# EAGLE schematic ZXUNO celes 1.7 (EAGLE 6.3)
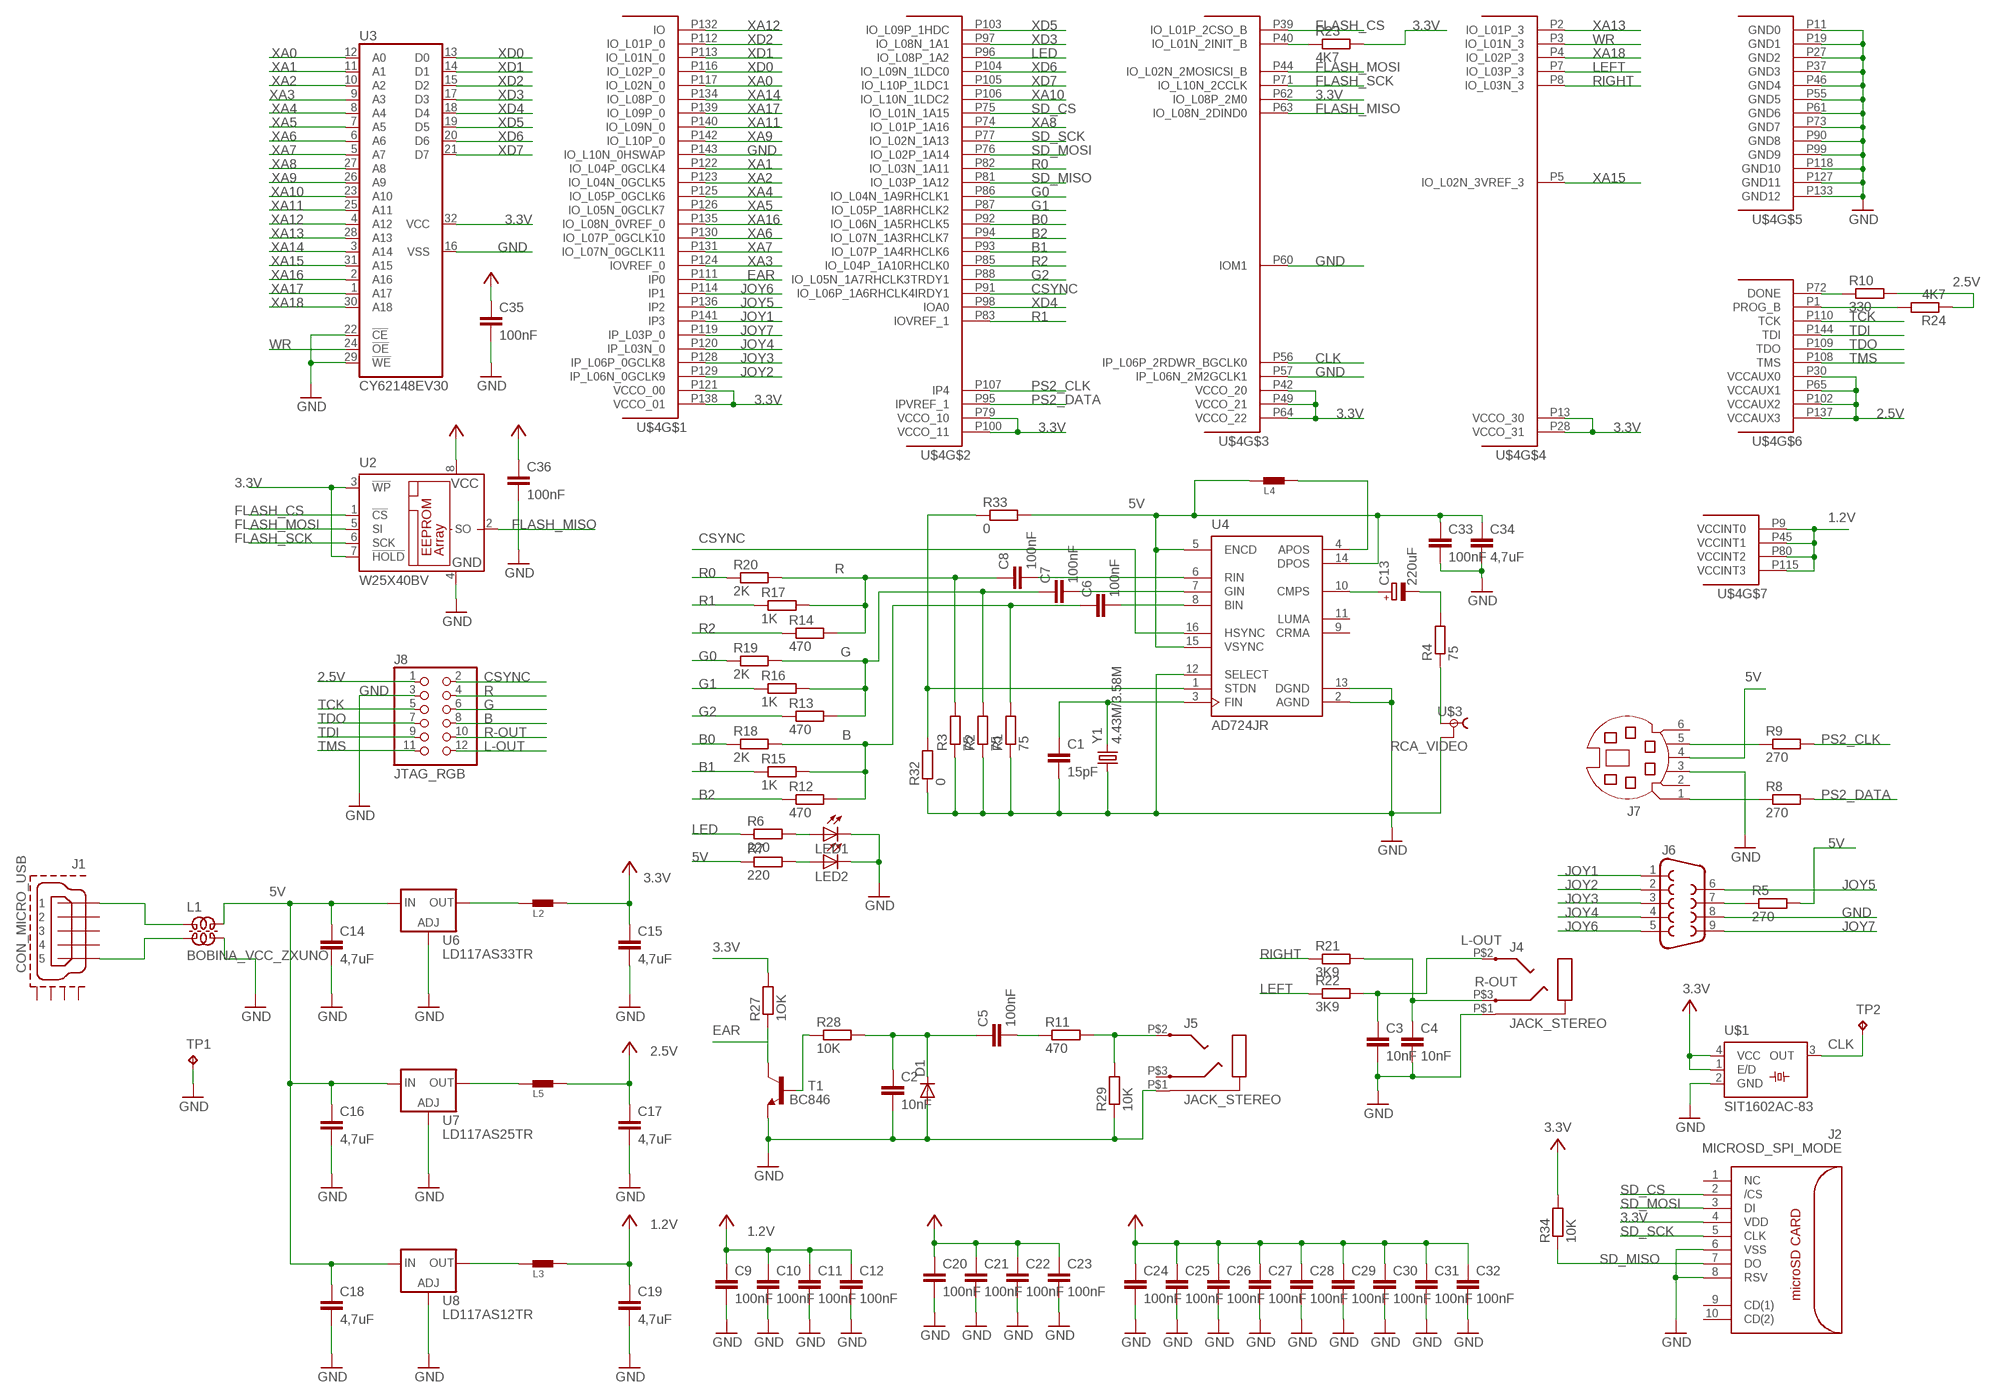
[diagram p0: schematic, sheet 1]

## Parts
C1  15pF  C-EUC0805  [C0805]
C2  10nF  C-EUC0805  [C0805]
C3  10nF  C-EUC0805  [C0805]
C4  10nF  C-EUC0805  [C0805]
C5  100nF  C-EUC0805  [C0805]
C6  100nF  C-EUC0805  [C0805]
C7  100nF  C-EUC0805  [C0805]
C8  100nF  C-EUC0805  [C0805]
C9  100nF  C-EUC0805  [C0805]
C10  100nF  C-EUC0805  [C0805]
C11  100nF  C-EUC0805  [C0805]
C12  100nF  C-EUC0805  [C0805]
C13  220uF  CPOL-EUE5-10.5  [E5-10,5]
C14  4,7uF  C-EUC0805  [C0805]
C15  4,7uF  C-EUC0805  [C0805]
C16  4,7uF  C-EUC0805  [C0805]
C17  4,7uF  C-EUC0805  [C0805]
C18  4,7uF  C-EUC0805  [C0805]
C19  4,7uF  C-EUC0805  [C0805]
C20  100nF  C-EUC0805  [C0805]
C21  100nF  C-EUC0805  [C0805]
C22  100nF  C-EUC0805  [C0805]
C23  100nF  C-EUC0805  [C0805]
C24  100nF  C-EUC0805  [C0805]
C25  100nF  C-EUC0805  [C0805]
C26  100nF  C-EUC0805  [C0805]
C27  100nF  C-EUC0805  [C0805]
C28  100nF  C-EUC0805  [C0805]
C29  100nF  C-EUC0805  [C0805]
C30  100nF  C-EUC0805  [C0805]
C31  100nF  C-EUC0805  [C0805]
C32  100nF  C-EUC0805  [C0805]
C33  100nF  C-EUC0805  [C0805]
C34  4,7uF  C-EUC0805  [C0805]
C35  100nF  C-EUC0805  [C0805]
C36  100nF  C-EUC0805  [C0805]
D1  DIODE-SOD123  [SOD123]
J1  CON_MICRO_USB  [MICRO_USB]
J2  MICROSD_SPI_MODE  [MICRO_SD_CONNECTOR]
J4  JACK_STEREO  [STX]
J5  JACK_STEREO  [STX]
J6  F09H  [F09H]
J7  MD06SS  [MDIN06SS]
J8  JTAG_RGB  PINHD-2X6/90  [2X06/90]
L1  BOBINA_VCC_ZXUNO  [CHOKE_COMM]
L2  FERRITE  [0805]
L3  FERRITE  [0805]
L4  FERRITE  [0805]
L5  FERRITE  [0805]
LED1  LEDCHIPLED_1206  [CHIPLED_1206]
LED2  LEDCHIPLED_1206  [CHIPLED_1206]
R1  75  R-EU_R0805  [R0805]
R2  75  R-EU_R0805  [R0805]
R3  75  R-EU_R0805  [R0805]
R4  75  R-EU_R0805  [R0805]
R5  270  R-EU_R0805  [R0805]
R6  220  R-EU_R0805  [R0805]
R7  220  R-EU_R0805  [R0805]
R8  270  R-EU_R0805  [R0805]
R9  270  R-EU_R0805  [R0805]
R10  330  R-EU_R0805  [R0805]
R11  470  R-EU_R0805  [R0805]
R12  470  R-EU_R0805  [R0805]
R13  470  R-EU_R0805  [R0805]
R14  470  R-EU_R0805  [R0805]
R15  1K  R-EU_R0805  [R0805]
R16  1K  R-EU_R0805  [R0805]
R17  1K  R-EU_R0805  [R0805]
R18  2K  R-EU_R0805  [R0805]
R19  2K  R-EU_R0805  [R0805]
R20  2K  R-EU_R0805  [R0805]
R21  3K9  R-EU_R0805  [R0805]
R22  3K9  R-EU_R0805  [R0805]
R23  4K7  R-EU_R0805  [R0805]
R24  4K7  R-EU_R0805  [R0805]
R27  1OK  R-EU_R0805  [R0805]
R28  10K  R-EU_R0805  [R0805]
R29  10K  R-EU_R0805  [R0805]
R32  0  R-EU_R0805  [R0805]
R33  0  R-EU_R0805  [R0805]
R34  10K  R-EU_R0805  [R0805]
T1  BC846  [SOT23]
TP1  TPTP20SQ  [TP20SQ]
TP2  TPTP20SQ  [TP20SQ]
U2  W25X40BV  25AA080SN  [SO-08]
U3  CY62148EV30  MEMORIAZXUNO  [SOIC32]
U4  AD724JR  [SO16W]
U6  LD117AS33TR  [SOT223]
U7  LD117AS25TR  [SOT223]
U8  LD117AS12TR  [SOT223]
U$1  SIT1602AC-83  [SM77H]
U$3  RCA_VIDEO  [RCA_PACK]
U$4  XILINXXC3S250ETQ1442CARAS  [TQ144_DIP_INCOMPLETO_2CARAS]
Y1  4.43M/3.58M  CRYSTALHC18U-V  [HC18U-V]

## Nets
1.2V: C9.1 C10.1 C11.1 C12.1 C19.1 L3.2 U$4.P9(VCCINT0) U$4.P45(VCCINT1) U$4.P80(VCCINT2) U$4.P115(VCCINT3) ; supply symbol labelled +3V3
2.5V [alimentacion]: C17.1 C20.1 C21.1 C22.1 C23.1 J8.1 L5.2 R10.2 R24.1 U$4.P30(VCCAUX0) U$4.P65(VCCAUX1) U$4.P102(VCCAUX2) U$4.P137(VCCAUX3) ; supply symbol labelled +3V3
3.3V [alimentacion]: C15.1 C24.1 C25.1 C26.1 C27.1 C28.1 C29.1 C30.1 C31.1 C32.1 C35.1 C36.1 J2.4(VDD) L2.2 R23.2 R27.2 R34.2 U2.3(!WP) U2.7(!HOLD) U2.8(VCC) U3.32(VCC) U$1.1(E/D) U$1.4(VCC) U$4.P13(VCCO_30) U$4.P28(VCCO_31) U$4.P42(VCCO_20) U$4.P49(VCCO_21) U$4.P62(IO_L08P_2M0) U$4.P64(VCCO_22) U$4.P79(VCCO_10) U$4.P100(VCCO_11) U$4.P121(VCCO_00) U$4.P138(VCCO_01) ; supply symbol labelled +3V3
5V [alimentacion]: C14.1 C16.1 C18.1 C33.1 C34.1 J7.4 L1.P$4 L4.1 R5.2 R7.1 R33.2 U4.5(ENCD) U4.14(DPOS) U4.15(VSYNC) U6.3(IN) U7.3(IN) U8.3(IN)
B: C6.1 J8.8 R1.2 R12.2 R15.2 R18.2
B0: R18.1 U$4.P92(IO_L06N_1A5RHCLK5)
B1: R15.1 U$4.P93(IO_L07P_1A4RHCLK6)
B2: R12.1 U$4.P94(IO_L07N_1A3RHCLK7)
CLK: TP2.TP U$1.3(OUT) U$4.P56(IP_L06P_2RDWR_BGCLK0)
CSYNC: J8.2 U4.16(HSYNC) U$4.P91(IO_L06P_1A6RHCLK4IRDY1)
EAR: R27.1 T1.3(C) U$4.P111(IP0)
FLASH_CS: U2.1(!CS) U$4.P39(IO_L01P_2CSO_B)
FLASH_MISO: U2.2(SO) U$4.P63(IO_L08N_2DIND0)
FLASH_MOSI: U2.5(SI) U$4.P44(IO_L02N_2MOSICSI_B)
FLASH_SCK: U2.6(SCK) U$4.P71(IO_L10N_2CCLK)
G: C7.1 J8.6 R2.2 R13.2 R16.2 R19.2
G0: R19.1 U$4.P86(IO_L04N_1A9RHCLK1)
G1: R16.1 U$4.P87(IO_L05P_1A8RHCLK2)
G2: R13.1 U$4.P88(IO_L05N_1A7RHCLK3TRDY1)
GND [alimentacion]: C1.2 C2.2 C3.2 C4.2 C9.2 C10.2 C11.2 C12.2 C14.2 C15.2 C16.2 C17.2 C18.2 C19.2 C20.2 C21.2 C22.2 C23.2 C24.2 C25.2 C26.2 C27.2 C28.2 C29.2 C30.2 C31.2 C32.2 C33.2 C34.2 C35.2 C36.2 D1.A J2.6(VSS) J2.8(RSV) J4.P$1 J5.P$1 J6.8 J7.3 J8.3 L1.P$3 LED1.C LED2.C R1.1 R2.1 R3.1 R29.1 R32.1 T1.2(E) TP1.TP U2.4(GND) U3.16(VSS) U3.22(!CE) U3.29(!WE) U4.2(AGND) U4.12(SELECT) U4.13(DGND) U6.1(ADJ) U7.1(ADJ) U8.1(ADJ) U$1.2(GND) U$3.1 U$4.P11(GND0) U$4.P19(GND1) U$4.P27(GND2) U$4.P37(GND3) U$4.P46(GND4) U$4.P55(GND5) U$4.P57(IP_L06N_2M2GCLK1) U$4.P60(IOM1) U$4.P61(GND6) U$4.P73(GND7) U$4.P90(GND8) U$4.P99(GND9) U$4.P118(GND10) U$4.P127(GND11) U$4.P133(GND12) U$4.P143(IO_L10N_0HSWAP) Y1.1
JOY1: J6.1 U$4.P141(IP3)
JOY2: J6.2 U$4.P129(IP_L06N_0GCLK9)
JOY3: J6.3 U$4.P128(IP_L06P_0GCLK8)
JOY4: J6.4 U$4.P120(IP_L03N_0)
JOY5: J6.6 U$4.P136(IP2)
JOY6: J6.5 U$4.P114(IP1)
JOY7: J6.9 U$4.P119(IP_L03P_0)
L-OUT: C3.1 J4.P$2 J8.12 R22.2
LED: R6.1 U$4.P96(IO_L08P_1A2)
LEFT: R22.1 U$4.P7(IO_L03P_3)
N$1: C8.2 U4.6(RIN)
N$2: C7.2 U4.7(GIN)
N$3: C6.2 U4.8(BIN)
N$4: R32.2 R33.1 U4.1(STDN)
N$5: LED1.A R6.2
N$6: C1.1 U4.3(FIN) Y1.2
N$7: C13.+ U4.10(CMPS)
N$8: LED2.A R7.2
N$9: C13.- R4.2
N$10: R4.1 U$3.2 U$3.2@1
N$11: R28.1 T1.1(B)
N$12: C2.1 C5.1 D1.C R28.2
N$13: C5.2 R11.1
N$14: J5.P$2 R11.2 R29.2
N$15: R24.2 U$4.P1(PROG_B)
N$16: R10.1 U$4.P72(DONE)
N$17: R23.1 U$4.P40(IO_L01N_2INIT_B)
N$18: J7.1 R8.1
N$19: J7.5 R9.1
N$20: J6.7 R5.1
N$21 [alimentacion]: L2.1 U6.2(OUT) U6.4(OUT)
N$22 [alimentacion]: L5.1 U7.2(OUT) U7.4(OUT)
N$23 [alimentacion]: L3.1 U8.2(OUT) U8.4(OUT)
N$24: L4.2 U4.4(APOS)
N$25 [alimentacion]: J1.1 L1.P$1
N$26 [alimentacion]: J1.5 L1.P$2
PS2_CLK: R9.2 U$4.P107(IP4)
PS2_DATA: R8.2 U$4.P95(IPVREF_1)
R: C8.1 J8.4 R3.2 R14.2 R17.2 R20.2
R0: R20.1 U$4.P82(IO_L03N_1A11)
R1: R17.1 U$4.P83(IOVREF_1)
R2: R14.1 U$4.P85(IO_L04P_1A10RHCLK0)
R-OUT: C4.1 J4.P$3 J8.10 R21.2
RIGHT: R21.1 U$4.P8(IO_L03N_3)
SD_CS: J2.2(/CS) U$4.P75(IO_L01N_1A15)
SD_MISO: J2.7(DO) R34.1 U$4.P81(IO_L03P_1A12)
SD_MOSI: J2.3(DI) U$4.P76(IO_L02P_1A14)
SD_SCK: J2.5(CLK) U$4.P77(IO_L02N_1A13)
TCK: J8.5 U$4.P110(TCK)
TDI: J8.9 U$4.P144(TDI)
TDO: J8.7 U$4.P109(TDO)
TMS: J8.11 U$4.P108(TMS)
WR: U3.24(!OE) U$4.P3(IO_L01N_3)
XA0: U3.12(A0) U$4.P117(IO_L02N_0)
XA1: U3.11(A1) U$4.P122(IO_L04P_0GCLK4)
XA2: U3.10(A2) U$4.P123(IO_L04N_0GCLK5)
XA3: U3.9(A3) U$4.P124(IOVREF_0)
XA4: U3.8(A4) U$4.P125(IO_L05P_0GCLK6)
XA5: U3.7(A5) U$4.P126(IO_L05N_0GCLK7)
XA6: U3.6(A6) U$4.P130(IO_L07P_0GCLK10)
XA7: U3.5(A7) U$4.P131(IO_L07N_0GCLK11)
XA8: U3.27(A8) U$4.P74(IO_L01P_1A16)
XA9: U3.26(A9) U$4.P142(IO_L10P_0)
XA10: U3.23(A10) U$4.P106(IO_L10N_1LDC2)
XA11: U3.25(A11) U$4.P140(IO_L09N_0)
XA12: U3.4(A12) U$4.P132(IO)
XA13: U3.28(A13) U$4.P2(IO_L01P_3)
XA14: U3.3(A14) U$4.P134(IO_L08P_0)
XA15: U3.31(A15) U$4.P5(IO_L02N_3VREF_3)
XA16: U3.2(A16) U$4.P135(IO_L08N_0VREF_0)
XA17: U3.1(A17) U$4.P139(IO_L09P_0)
XA18: U3.30(A18) U$4.P4(IO_L02P_3)
XD0: U3.13(D0) U$4.P116(IO_L02P_0)
XD1: U3.14(D1) U$4.P113(IO_L01N_0)
XD2: U3.15(D2) U$4.P112(IO_L01P_0)
XD3: U3.17(D3) U$4.P97(IO_L08N_1A1)
XD4: U3.18(D4) U$4.P98(IOA0)
XD5: U3.19(D5) U$4.P103(IO_L09P_1HDC)
XD6: U3.20(D6) U$4.P104(IO_L09N_1LDC0)
XD7: U3.21(D7) U$4.P105(IO_L10P_1LDC1)
Unconnected: J1.2 J1.3 J1.4 J1.P$1(GND1) J1.P$2(GND2) J1.P$3(GND3) J1.P$4(GND4) J2.1(NC) J2.9(CD(1)) J2.10(CD(2)) J5.P$3 J7.2 J7.6 U4.9(CRMA) U4.11(LUMA)

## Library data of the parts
C1-C12 C14-C36 = rcl:C-EU: CAPACITOR, European symbol
C13 = rcl:CPOL-EU: POLARIZED CAPACITOR, European symbol
D1 = diode:DIODE-: DIODE
J1 = ZXUNO:CON_MICRO_USB
J2 = con-molex-microsd:MICROSD_SPI_MODE: MOLEX - 49225-0821 - CONNECTEUR MICRO SD PUSH/PUSH REV Fabricant: MOLEX Code commande Farnell: 1366700 Référence fabricant: 49225-0821
J4 J5 = ZXUNO:JACK_STEREO
J6 = con-subd:F09: SUB-D; OC_FARNELL: unknown; OC_NEWARK: unknown
J7 = con-yamaichi:MD06SS: YAMAICHI CONNECTOR; OC_FARNELL: unknown; OC_NEWARK: unknown
J8 = pinhead:PINHD-2X6: PIN HEADER
L1 = ZXUNO:BOBINA_VCC_ZXUNO
L2-L5 = Murata AWJLEagleLib:FERRITE: Ferrite bead
LED1 LED2 = led:LED: LED
R1-R24 R27-R29 R32-R34 = rcl:R-EU_: RESISTOR, European symbol
T1 = transistor:BC846: NPN TRANSISTOR
TP1 TP2 = testpad:TP: Test pad
U2 = microchip:25*: Serial EEPROM 4K/ 8K , SPI bus; MF: MICROCHIP; MPN: 25AA080/SN; OC_FARNELL: 1816072; OC_NEWARK: 92C7351
U3 = ZXUNO:MEMORIAZXUNO
U4 = vga2tv:AD724
U6-U8 = v-reg:LD117A?*: Low drop fixed and adjustable positive voltage regulators 1 A Source: http://www.st.com/stonline/products/literature/ds/7194/ld1117axx.pdf
U$1 = ZXUNO:SIT1602AC-83
U$3 = ZXUNO:RCA_VIDEO
U$4 = xilinx_spartan3_virtex4_and_5:XILINXXC3S250ETQ144
Y1 = crystal:CRYSTAL: CRYSTAL; OC_FARNELL: unknown; OC_NEWARK: unknown

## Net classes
0 default: width 0.381 mm, drill 0.203 mm, clearance 0.203 mm
1 alimentacion: width 0.508 mm, drill 0.203 mm, clearance 0.203 mm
